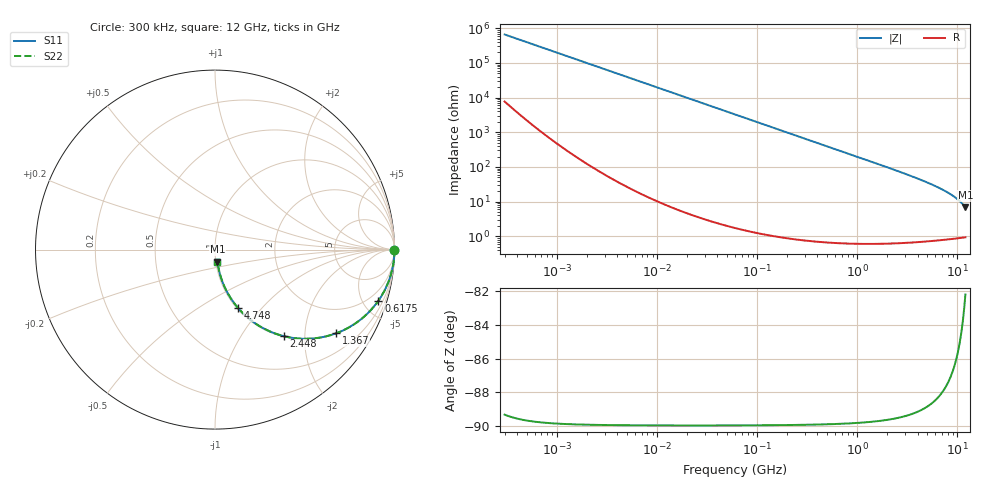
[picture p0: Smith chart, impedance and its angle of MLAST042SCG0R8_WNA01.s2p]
! MLAST042SCG0R8_WNA01  S-PARAMETER MODEL  ( General Type )
! Model Generated by TAIYO YUDEN Corporation (http://www.ty-top.com)
! Version 1.0
! TAIYO YUDEN Control No. 150820
! Copyright(c) 2015 TAIYO YUDEN CO.,LTD. All Rights Reserved.
! Product Description (link to TY-COMPAS)
! https://ds.yuden.co.jp/TYCOMPAS/or/detail?pn=MLAST042SCG0R8AWNA01&u=M
! Products Name : Multilayer Ceramic Capacitors
! Characteristics :
!  Capacitance : 0.8 pF , Rated Voltage : 25V , TCC : CG / C0G
!  Case Size : 0.4 x 0.2 / 0.016 x 0.008 [mm/inch] , Thickness : 0.2 / 0.008 [mm/inch]
!  (Conditions: Temperature = 25 degC , DC Bias Current/Voltage = 0A / 0V)
! External Node Assignments :
!  1  o---| |---o  2
! GND o---------o GND
! Frequency Range : 0.3MHz  -  12000MHz  [ 401 STEP ]
# MHz S RI R 50
! Freq[MHz].  S11 Real  S11 Imag  S21 Real  S21 Imag  S12 Real  S12 Imag  S22 Real  S22 Imag
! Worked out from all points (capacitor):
!   401 points, 300 kHz to 12 GHz, reference 50 ohm
!   read as one part in series: C = 803 fF near 316.3 kHz
!   lowest |Z| = 6.88 ohm at 12 GHz (marker M1)
!   S11 on the Smith chart (normalised r, x): 300 kHz: open; 617.5 MHz: 1.01, -6.41; 1.367 GHz: 1.01, -2.88; 2.448 GHz: 1.01, -1.58; 4.748 GHz: 1.01, -0.76; 12 GHz: 1.02, -0.14
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0.3  1 -0.000151  1.79e-06 0.000151  1.79e-06 0.000151  1 -0.000151
1.769972  1 -0.000893  2.01e-06 0.000893  2.01e-06 0.000893  1 -0.000893
10.44266  1 -0.00527  3.04e-05 0.00527  3.04e-05 0.00527  1 -0.00527
60  0.9991 -0.0302  0.000931 0.0302  0.000931 0.0302  0.9991 -0.0302
164.1901  0.9931 -0.0823  0.00688 0.0823  0.00688 0.0823  0.9931 -0.0823
244.3004  0.9849 -0.1214  0.0151 0.1214  0.0151 0.1214  0.9849 -0.1214
353.9943  0.9689 -0.1731  0.0311 0.1731  0.0311 0.1731  0.9689 -0.1731
473.7541  0.9456 -0.2261  0.0544 0.2261  0.0544 0.2261  0.9456 -0.2261
617.4538  0.9108 -0.284  0.0892 0.284  0.0892 0.284  0.9108 -0.284
918.7169  0.8215 -0.3815  0.1785 0.3815  0.1785 0.3815  0.8215 -0.3815
1105.905  0.7601 -0.4253  0.2399 0.4253  0.2399 0.4253  0.7601 -0.4253
1366.97  0.6737 -0.4668  0.3263 0.4668  0.3263 0.4668  0.6737 -0.4668
1689.663  0.5731 -0.492  0.4269 0.492  0.4269 0.492  0.5731 -0.492
2088.533  0.4652 -0.4955  0.5348 0.4955  0.5348 0.4955  0.4652 -0.4955
2448.343  0.3851 -0.4827  0.6149 0.4827  0.6149 0.4827  0.3851 -0.4827
3454.93  0.2323 -0.4163  0.7677 0.4163  0.7677 0.4163  0.2323 -0.4163
4747.894  0.1303 -0.3274  0.8697 0.3274  0.8697 0.3274  0.1303 -0.3274
6524.734  0.0656 -0.2328  0.9344 0.2328  0.9344 0.2328  0.0656 -0.2328
8281.503  0.0363 -0.1648  0.9637 0.1648  0.9637 0.1648  0.0363 -0.1648
9968.853  0.0221 -0.1146  0.9779 0.1146  0.9779 0.1146  0.0221 -0.1146
11380.75  0.0156 -0.0801  0.9844 0.0801  0.9844 0.0801  0.0156 -0.0801
12000  0.0138 -0.0666  0.9862 0.0666  0.9862 0.0666  0.0138 -0.0666
